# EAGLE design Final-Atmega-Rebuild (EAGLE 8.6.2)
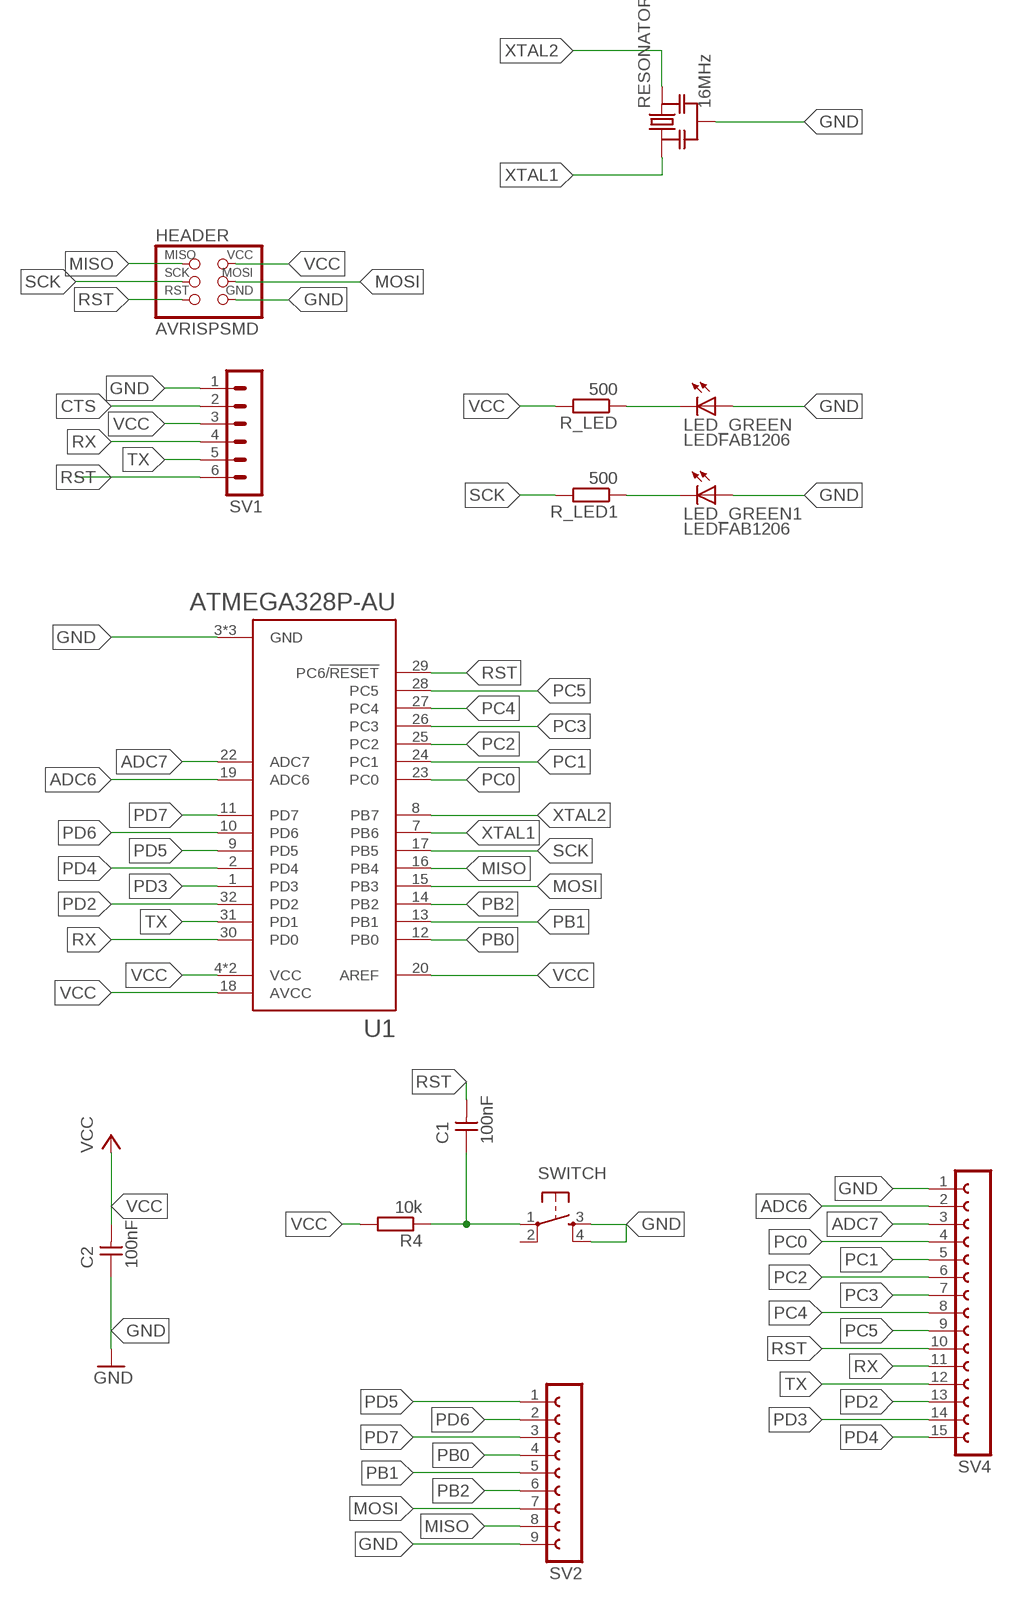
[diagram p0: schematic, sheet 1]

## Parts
C1  100nF  CAP-UNPOLARIZEDFAB  [C1206FAB]
C2  100nF  CAP-UNPOLARIZEDFAB  [C1206FAB]
HEADER  AVRISPSMD  [2X03SMD]
LED_GREEN  LEDFAB1206  [LED1206FAB]
LED_GREEN1  LEDFAB1206  [LED1206FAB]
R4  10k  R-EU_R1206  [R1206]
R_LED  500  R-EU_R1206  [R1206]
R_LED1  500  R-EU_R1206  [R1206]
RESONATOR  16MHz  RESONATOR-MURATACSTCR_G  [RESONATOR_MURATA3]
SV1  MA06-1  [MA06-1]
SV2  FE09-1  [FE09]
SV4  FE15-1  [FE15]
SWITCH  6MM_SWITCH6MM_SWITCH  [6MM_SWITCH]
U1  ATMEGA328P-AU  [QFP80P900X900X120-32N]

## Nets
ADC6: SV4.2 U1.19(ADC6)
ADC7: SV4.3 U1.22(ADC7)
CTS: SV1.2
GND: C2.1 HEADER.6(GND) LED_GREEN1.1(A) LED_GREEN.1(A) RESONATOR.2 SV1.1 SV4.1 SWITCH.3(S) SWITCH.4(S1) U1.3(GND) U1.5(GND) U1.21(GND)
MISO: HEADER.1(MISO) SV2.8 U1.16(PB4)
MOSI: HEADER.4(MOSI) SV2.7 U1.15(PB3)
N$1: LED_GREEN1.2(C) R_LED1.1
N$21: LED_GREEN.2(C) R_LED.1
PB0: SV2.4 U1.12(PB0)
PB1: SV2.5 U1.13(PB1)
PB2: SV2.6 U1.14(PB2)
PC0: SV4.4 U1.23(PC0)
PC1: SV4.5 U1.24(PC1)
PC2: SV4.6 U1.25(PC2)
PC3: SV4.7 U1.26(PC3)
PC4: SV4.8 U1.27(PC4)
PC5: SV4.9 U1.28(PC5)
PD2: SV4.13 U1.32(PD2)
PD3: SV4.14 U1.1(PD3)
PD4: SV4.15 U1.2(PD4)
PD5: SV2.1 U1.9(PD5)
PD6: SV2.2 U1.10(PD6)
PD7: SV2.3 U1.11(PD7)
RST: C1.1 C1.2 HEADER.5(RST) R4.1 SV1.6 SV4.10 SWITCH.1(P) U1.29(PC6/!RESET)
RX: SV1.4 SV4.11 U1.30(PD0)
SCK: HEADER.3(SCK) R_LED1.2 U1.17(PB5)
TX: SV1.5 SV4.12 U1.31(PD1)
VCC: C2.2 HEADER.2(VCC) R4.2 R_LED.2 SV1.3 U1.4(VCC) U1.6(VCC) U1.18(AVCC) U1.20(AREF)
XTAL1: RESONATOR.1 U1.7(PB6)
XTAL2: RESONATOR.3 U1.8(PB7)
Unconnected: SV2.9 SWITCH.2(P1)

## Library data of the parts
C1 C2 = fab:CAP-UNPOLARIZED
HEADER = fab:AVRISP
LED_GREEN LED_GREEN1 = fab:LED: LED
R4 R_LED R_LED1 = resistor:R-EU_: RESISTOR, European symbol
RESONATOR = m-pad-2.1:RESONATOR-MURATA: Murata ceramic Resonator "ceralock" CSTCE series with built in load capacitance +- 0.5% tolerance 12.51MHz to 19.99MHz 16MHz murata part#: CSTCE16M0V53-R0 16MHz digikey part#: 490-1198-1-ND $1.33 each
SV1 = con-lstb:MA06-1: PIN HEADER; OC_FARNELL: unknown; OC_NEWARK: unknown
SV2 = con-lsta:FE09-1: FEMALE HEADER; OC_FARNELL: unknown; OC_NEWARK: unknown
SV4 = con-lsta:FE15-1: FEMALE HEADER; OC_FARNELL: unknown; OC_NEWARK: unknown
SWITCH = fab:6MM_SWITCH: OMRON SWITCH
U1 = ATMEGA328P-AU:ATMEGA328P-AU: ATmega Series 20 MHz 32 KB Flash 2 KB SRAM 8-Bit Microcontroller - TQFP-32; AVAILABILITY: Good; DESCRIPTION: ATmega Series 20 MHz 32 KB Flash 2 KB SRAM 8-Bit Microcontroller - TQFP-32; MF: Atmel; MP: ATMEGA328P-AU; PACKAGE: TQFP-32 Atmel; PRICE: 2.38 USD

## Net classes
0 default: clearance 0.205 mm

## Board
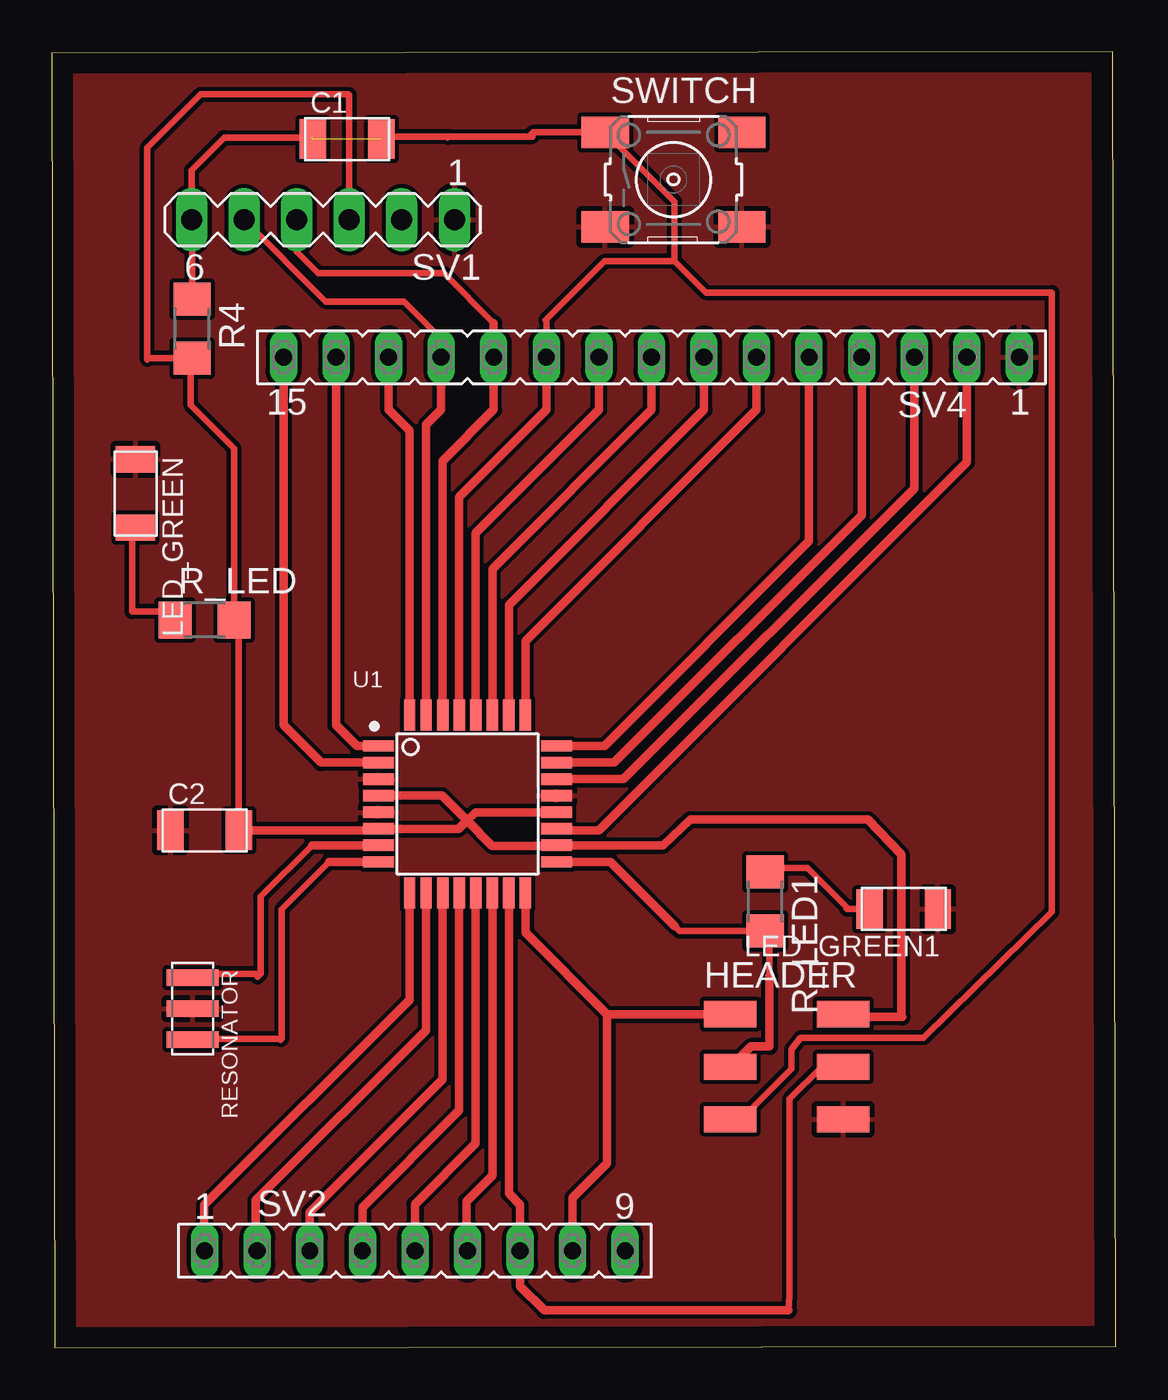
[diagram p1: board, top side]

Size 51.43 x 62.63 mm. Coordinates in mm from the lower left corner, seen from the top.
Outline: 0.14,0 51.43,0.08 51.29,62.63 0,62.54 0.14,0
Copper layers (1*16): Top 0.035mm / dielectric 1.5mm / Bottom 0.035mm
Design rules "default *": minimum track width 6mil, minimum drill 0.35mm, track to track 8mil, track to pad 8mil, pad to pad 8mil, via to via 8mil, smd to smd 8mil, copper to edge 40mil, drill to drill 8mil, minimum pad ring 10mil, minimum via ring 8mil, stop-mask expansion 4mil, vias tented up to drill 0mil, thermal gap 10mil

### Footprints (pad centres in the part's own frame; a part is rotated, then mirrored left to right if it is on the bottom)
C1206FAB = smd 1.27 x 1.905: 1 -1.651,0; 2 1.651,0
2X03SMD = smd 2.54 x 1.27: 1 -2.54,2.54; 2 2.92,2.54; 3 -2.54,0; 4 2.92,0; 5 -2.54,-2.54; 6 2.92,-2.54
LED1206FAB = smd 1.27 x 1.905: 1 -1.651,0; 2 1.651,0
R1206 = smd 1.6 x 1.803: 1 -1.422,0; 2 1.422,0
RESONATOR_MURATA3 = smd 0.8 x 2.5: 1 -1.5,0; 2 0,0; 3 1.5,0
MA06-1 = drill 1.016 long: 1 -6.35,0; 2 -3.81,0; 3 -1.27,0; 4 1.27,0; 5 3.81,0; 6 6.35,0
FE09 = drill 0.813 long: 1 -10.16,0; 2 -7.62,0; 3 -5.08,0; 4 -2.54,0; 5 0,0; 6 2.54,0; 7 5.08,0; 8 7.62,0; 9 10.16,0
FE15 = drill 0.813 long: 1 -17.78,0; 2 -15.24,0; 3 -12.7,0; 4 -10.16,0; 5 -7.62,0; 6 -5.08,0; 7 -2.54,0; 8 0,0; 9 2.54,0; 10 5.08,0; 11 7.62,0; 12 10.16,0; 13 12.7,0; 14 15.24,0; 15 17.78,0
6MM_SWITCH = smd 2.286 x 1.524: 1 -3.302,2.286; 2 3.302,2.286; 3 -3.302,-2.286; 4 3.302,-2.286
QFP80P900X900X120-32N = smd 1.5 x 0.55: 1 -4.3,2.8; 2 -4.3,2; 3 -4.3,1.2; 4 -4.3,0.4; 5 -4.3,-0.4; 6 -4.3,-1.2; 7 -4.3,-2; 8 -4.3,-2.8; 17 4.3,-2.8; 18 4.3,-2; 19 4.3,-1.2; 20 4.3,-0.4; 21 4.3,0.4; 22 4.3,1.2; 23 4.3,2; 24 4.3,2.8 | smd 0.55 x 1.5: 9 -2.8,-4.3; 10 -2,-4.3; 11 -1.2,-4.3; 12 -0.4,-4.3; 13 0.4,-4.3; 14 1.2,-4.3; 15 2,-4.3; 16 2.8,-4.3; 25 2.8,4.3; 26 2,4.3; 27 1.2,4.3; 28 0.4,4.3; 29 -0.4,4.3; 30 -1.2,4.3; 31 -2,4.3; 32 -2.8,4.3

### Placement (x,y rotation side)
C1  14.27,58.41 0 top
C2  7.39,25.01 0 top
HEADER  35.33,13.58 0 top
LED_GREEN  4.05,41.28 270 top
LED_GREEN1  41.17,21.2 180 top
R4  6.79,49.25 270 top
R_LED  7.39,35.17 0 top
R_LED1  34.47,21.56 270 top
RESONATOR  6.81,16.39 270 top
SV1  13.11,54.51 180 top
SV2  17.55,4.69 0 top
SV4  28.98,47.87 180 top
SWITCH  30.05,56.45 0 top
U1  20.09,26.28 0 top

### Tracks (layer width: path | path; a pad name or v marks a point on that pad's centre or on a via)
ADC6
  Top 0.406: U1.19 24.46,25.01 26.44,25.01 44.22,42.79 SV4.2
ADC7
  Top 0.406: U1.22 27.64,27.48 41.68,41.52 SV4.3
GND
  pour Top: -45.95,83.43 -45.95,-52.46 -44.68,-53.73 70.89,-53.73 77.24,-47.38 77.24,84.7 67.08,94.86 -34.52,94.86
MISO
  Top 0.406: U1.16 22.89,20.07 26.84,16.12 | 26.84,16.12 HEADER.1 | 26.84,16.12 26.84,8.91 25.17,7.24 SV2.8
MOSI
  Top 0.305: HEADER.4 37.21,13.58 35.65,12.02 35.65,2.51 35.61,1.8
  Top 0.406: HEADER.4 38.26,13.57 | 35.61,1.8 23.81,1.8 22.63,2.98 SV2.7 22.64,6.9 22.09,7.45 U1.15
N$1
  Top 0.305: R_LED1.1 34.67,23.18 36.52,23.18 38.41,21.3 38.41,21.22 38.43,21.2 LED_GREEN1.2
N$21
  Top 0.305: R_LED.1 5.57,35.57 3.88,35.57 3.88,39.46 LED_GREEN.2
  Top 0.406: R_LED.1 6.12,35.32
PB0
  Top 0.406: U1.12 19.69,11.46 15.03,6.8 15.03,4.7 SV2.4
PB1
  Top 0.406: U1.13 20.49,9.88 17.55,6.94 SV2.5
PB2
  Top 0.406: U1.14 21.29,8.33 20.04,7.08 20.04,4.74 SV2.6
PC0
  Top 0.406: U1.23 27.17,28.28 39.14,40.25 SV4.4
PC1
  Top 0.406: U1.24 26.7,29.08 36.6,38.98 SV4.5
PC2
  Top 0.406: U1.25 22.89,34.16 34.06,45.33 SV4.6
PC3
  Top 0.406: U1.26 22.09,35.9 31.52,45.33 SV4.7
PC4
  Top 0.406: U1.27 21.29,37.64 28.98,45.33 SV4.8
PC5
  Top 0.406: U1.28 20.49,39.38 26.44,45.33 SV4.9
PD2
  Top 0.406: U1.32 17.29,44.32 16.28,45.33 SV4.13
PD3
  Top 0.406: U1.1 14.75,29.08 13.74,30.09 SV4.14
PD4
  Top 0.406: U1.2 13.01,28.28 11.2,30.09 SV4.15
PD5
  Top 0.406: U1.9 17.29,16.82 7.37,6.9 7.37,4.71 SV2.1
PD6
  Top 0.406: U1.10 18.09,15.34 9.87,7.12 9.87,4.75 SV2.2
PD7
  Top 0.406: U1.11 18.89,12.98 12.47,6.56 SV2.3
RST  (2 unrouted)
  Top 0.305: 6.79,54.48 SV1.6 6.76,54.64 | 6.76,54.64 6.76,56.91 8.33,58.48 12.55,58.48 | 19.13,58.48 19.19,58.53 | 19.19,58.53 23.05,58.53 | 23.05,58.53 23.23,58.53 | 30.1,52.5 30.1,55.39 SWITCH.1 23.26,58.74 23.05,58.53 | 30.1,52.5 26.72,52.5 23.87,49.65 23.9,49.62 SV4.10 | 30.1,52.5 31.6,51 48.34,51 48.34,21.06 42.13,14.98 36.19,14.98 35.76,14.42 35.76,13.48 33.31,11.04 HEADER.5 | 19.19,58.53 16.05,58.53 C1.2 | R4.1 6.79,54.61 6.76,54.64
  Top 0.406: U1.29 19.69,41.12 23.9,45.33 SV4.10
RX
  Top 0.305: 21.36,49.52 18.96,51.92 12.88,51.92 11.84,52.96 SV1.4
  Top 0.406: U1.30 18.89,42.86 21.36,45.33 SV4.11 21.36,49.52
SCK
  Top 0.305: 30.12,20.35 30.33,20.14 R_LED1.2 34.69,19.93 34.69,17.97
  Top 0.406: U1.17 26.99,23.48 30.12,20.35 | HEADER.3 32.8,13.57 33.79,14.56 34.69,14.56 34.69,17.97
TX
  Top 0.305: SV4.12 18.82,48.76 17.02,50.56 13.25,50.56 SV1.5
  Top 0.406: SV4.12 18.82,45.33 18.09,44.6 U1.31
VCC
  Top 0.305: C2.2 9.04,34.94 R_LED.2 8.81,43.46 6.72,45.56 6.72,47.75 R4.2 4.69,47.82 4.62,47.76 4.62,58 7.2,60.57 14.35,60.57 14.38,60.54 SV1.3
  Top 0.406: U1.4 18.86,26.68 20.07,25.47 | 20.07,25.47 21.28,24.26 24.37,24.26 U1.18 29.55,24.28 30.87,25.53 39.44,25.53 41.05,23.85 41.05,16.04 41.1,15.99 38.38,15.99 HEADER.2 | 20.07,25.47 19.67,25.08 U1.6 15.72,25.01 C2.2 | U1.20 20.47,25.88 20.07,25.47
XTAL1
  Top 0.305: 12.57,24.28 10.09,21.8 10.09,18.06 | 10.09,18.06 9.95,17.91 | 10.09,18.06 6.98,18.06 RESONATOR.1
  Top 0.406: U1.7 12.57,24.28
XTAL2
  Top 0.305: 13.41,23.48 11.11,21.18 11.11,14.94 | 11.11,14.94 11.06,14.89 | 11.11,14.94 6.86,14.94 RESONATOR.3
  Top 0.406: U1.8 13.41,23.48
